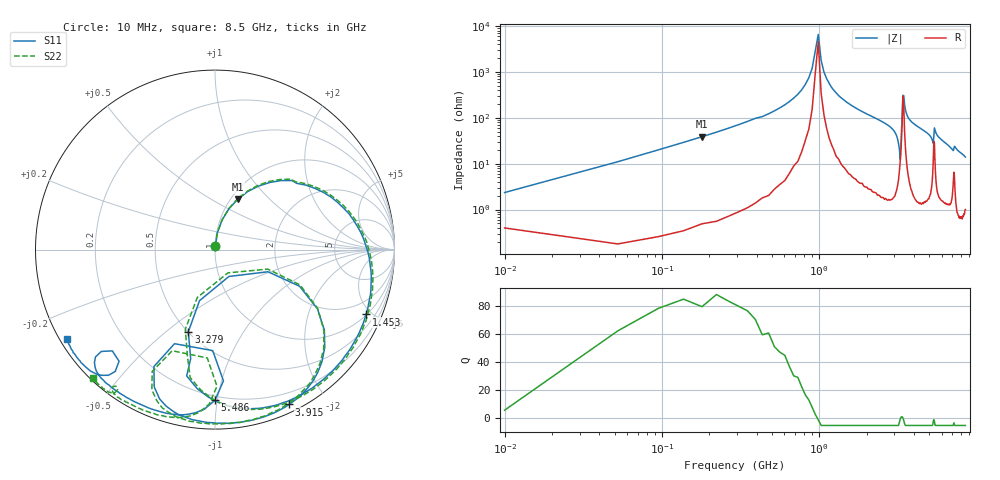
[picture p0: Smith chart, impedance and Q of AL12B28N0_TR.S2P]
!AVX CORPORATION
!PART NUMBER AL12B28N0_TR
!DESCRIPTION: AIR CORE INDUCTOR, 28nH, 8 TURNS
!Agilent Technologies,E5071C,MY46102230,A.09.54
!Date: Mon Sep 03 16:00:18 2012
!Data & Calibration Information:
!Freq	S11:SOLT2(ON)	S21:SOLT2(ON)	S12:SOLT2(ON)	S22:SOLT2(ON)
# Hz S RI R 50
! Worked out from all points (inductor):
!   201 points, 10 MHz to 8.5 GHz, reference 50 ohm
!   read as 1/Y11, port 2 shorted: L = 33.2 nH near 52.45 MHz
!   highest Q = 83.2 at 179.8 MHz (marker M1), where L = 34.3 nH
!   self-resonance near 943.9 MHz
!   S11 on the Smith chart (normalised r, x): 10 MHz: 1.00, +0.04; 1.453 GHz: 1.03, -4.64; 3.279 GHz: 0.50, -0.60; 3.915 GHz: 0.08, -1.58; 5.486 GHz: 0.17, -0.98; 8.5 GHz: 0.02, -0.28
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1e7  0.00119 0.0186  0.9985 -0.0238  0.9861 -0.0304  0.00127 0.0189
5.245e7  0.0135 0.0943  0.9859 -0.1223  0.9862 -0.1228  0.0134 0.0947
1.798e8  0.1278 0.2812  0.8681 -0.3759  0.8698 -0.3766  0.1257 0.2836
7.741e8  0.7709 0.1657  0.1403 -0.5834  0.1398 -0.584  0.7682 0.1846
1.4533e9  0.8418 -0.3613  -0.1362 -0.3407  -0.1364 -0.3409  0.8565 -0.3399
2.85415e9  0.235 -0.8849  -0.3292 -0.0847  -0.3292 -0.0844  0.2416 -0.8896
3.10885e9  -0.0387 -0.8207  -0.4898 0.0452  -0.4899 0.0455  -0.0251 -0.8254
3.27865e9  -0.1486 -0.4577  -0.6247 0.4163  -0.625 0.4168  -0.1655 -0.4443
3.36355e9  0.0777 -0.1496  -0.3616 0.7445  -0.3611 0.7449  0.0719 -0.1295
3.4909e9  0.5705 -0.3294  0.1788 0.5755  0.179 0.5753  0.5723 -0.3283
3.9154e9  0.4127 -0.8629  0.1597 0.0843  0.1599 0.0842  0.3781 -0.8775
4.255e9  0.2357 -0.9423  0.1112 0.027  0.1111 0.027  0.1857 -0.9517
4.89175e9  -0.0779 -0.9569  0.1061 -0.018  0.106 -0.0181  -0.1195 -0.9588
5.2738e9  -0.3387 -0.7651  0.1957 -0.1897  0.1957 -0.1896  -0.3517 -0.7811
5.3587e9  -0.2255 -0.5242  0.0494 -0.4128  0.0495 -0.4128  -0.2383 -0.5634
5.48605e9  -0.000438 -0.8394  -0.2122 -0.0962  -0.2122 -0.0961  -0.0327 -0.8612
5.6983e9  -0.2193 -0.919  -0.0773 0.0025  -0.0774 0.00253  -0.2314 -0.9344
6.58975e9  -0.5663 -0.7753  -0.0126 0.00746  -0.0124 0.00753  -0.4963 -0.8492
7.09915e9  -0.666 -0.5981  0.00043 0.0569  0.000468 0.0568  -0.5754 -0.776
7.2265e9  -0.5345 -0.6221  0.0864 0.0344  0.0864 0.0344  -0.5426 -0.7791
7.8208e9  -0.7509 -0.6215  0.023 -0.02  0.0231 -0.0196  -0.6341 -0.766
8.5e9  -0.8228 -0.4987  0.0314 -0.0327  0.0318 -0.0326  -0.6823 -0.7141
